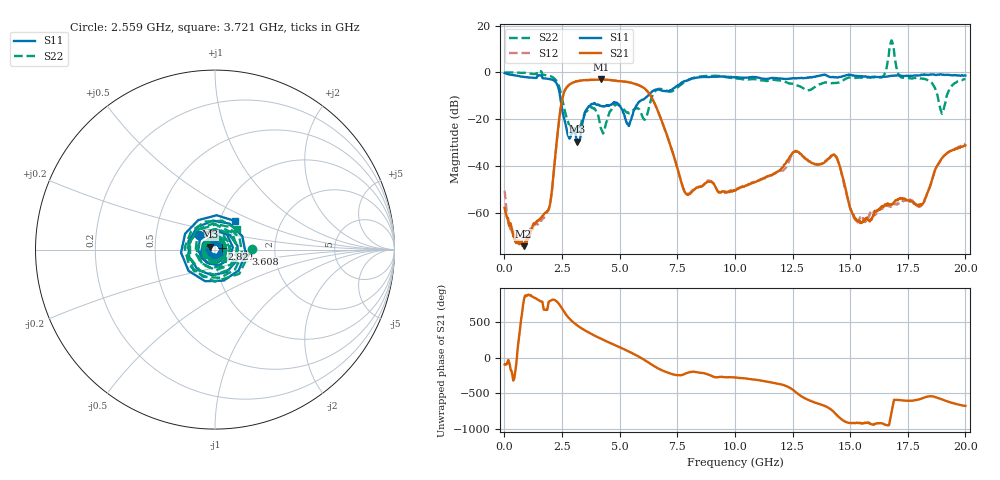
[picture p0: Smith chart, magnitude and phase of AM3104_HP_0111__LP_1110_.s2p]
!Created with skrf (http://scikit-rf.org).
# Hz S RI R 50.0
!freq ReS11 ImS11 ReS21 ImS21 ReS12 ImS12 ReS22 ImS22
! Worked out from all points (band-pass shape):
!   1601 points, 10 MHz to 20 GHz, reference 50 ohm
!   highest |S21| = -3.07 dB at 4.183 GHz (marker M1); lowest = -74.3 dB at 834.6 MHz (marker M2)
!   |S21| within 3 dB of the highest: 2.733 GHz to 5.947 GHz (3.214 GHz wide, 74.1 % of centre)
!   lowest |S11| = -29.7 dB at 3.171 GHz (marker M3), VSWR 1.07, Z = 47.2 + j1.56 ohm
!   |S11| at or under -10 dB: 2.413 GHz to 6.221 GHz (3.808 GHz wide, 88.2 % of centre)
!   |S22| runs from -26.2 to 13.6 dB; largest |S21 - S12| = 0.077
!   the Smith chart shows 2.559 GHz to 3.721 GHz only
!   S11 on the Smith chart (normalised r, x): 2.559 GHz: 0.83, +0.13; 2.821 GHz: 1.08, +0.01; 3.608 GHz: 1.41, -0.07; 3.721 GHz: 1.19, +0.39
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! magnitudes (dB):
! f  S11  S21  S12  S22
! 10 MHz  -0.3  -57.9  -50.6  -0.1
! 259.9 MHz  -1.0  -64.4  -67.0  -0.1
! 834.6 MHz  -2.0  -74.3  -70.1  -0.2
! 1.934 GHz  -2.8  -58.0  -58.2  -1.4
! 2.559 GHz  -18.5  -9.5  -9.5  -13.8
! 2.821 GHz  -28.3  -5.3  -5.3  -22.7
! 3.171 GHz  -29.7  -3.8  -3.8  -25.3
! 3.346 GHz  -24.1  -3.5  -3.5  -21.6
! 3.608 GHz  -15.3  -3.3  -3.4  -16.2
! 3.721 GHz  -14.2  -3.2  -3.3  -15.5
! 4.183 GHz  -14.4  -3.1  -3.1  -23.8
! 5.395 GHz  -22.9  -4.2  -4.3  -17.5
! 6.682 GHz  -7.3  -17.1  -17.1  -7.1
! 7.881 GHz  -3.7  -51.9  -51.6  -3.8
! 10.01 GHz  -2.2  -50.6  -50.2  -2.7
! 13.34 GHz  -2.2  -38.8  -38.7  -7.2
! 14.37 GHz  -2.1  -35.8  -36.0  -4.5
! 15.36 GHz  -1.8  -63.8  -62.9  -2.3
! 16.68 GHz  -1.6  -56.4  -57.0  7.3
! 18.11 GHz  -1.0  -56.7  -56.6  -2.7
! 18.98 GHz  -1.0  -36.8  -36.8  -17.6
! 20 GHz  -1.4  -31.2  -30.6  -2.9
